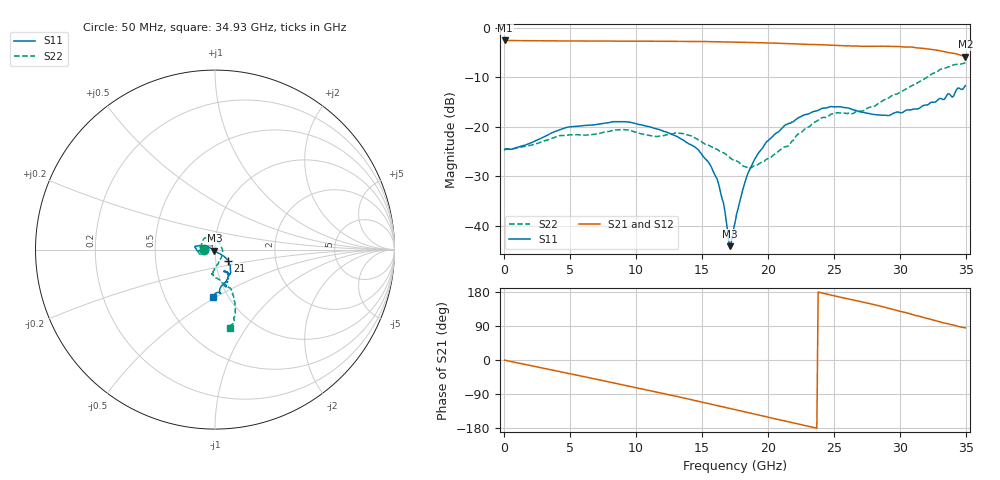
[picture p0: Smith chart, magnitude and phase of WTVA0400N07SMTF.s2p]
! 50 ohm 2-Port S-parameters measured by Modelithics Inc support@modelithics.com  Tampa, FL USA 813-866-6335 (February 2024)
! Smiths Interconnect,  4dB P/N: WTVA0400N07SMTF, Temperature: 125 C
! Board: 10 mil Rogers 4350B, Mounting Pad Dimensions: Length: 15 mils, Width: 25 mils, Gap: 40 mils.
# Hz S RI R 50
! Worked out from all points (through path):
!   352 points, 50 MHz to 34.93 GHz, reference 50 ohm
!   highest |S21| = -2.54 dB at 100 MHz (marker M1); lowest = -5.8 dB at 34.93 GHz (marker M2)
!   group delay of S21, straight-line fit = 21.8 ps
!   lowest |S11| = -44.1 dB at 17.11 GHz (marker M3), VSWR 1.01, Z = 49.6 - j0.508 ohm
!   |S11| at or under -10 dB: start of sweep to end of sweep
!   |S22| runs from -28.4 to -7.0 dB; largest |S21 - S12| = 0.0081
!   S11 on the Smith chart (normalised r, x): 50 MHz: 0.89, +0.00; 21 GHz: 1.15, -0.14; 34.93 GHz: 0.86, -0.48
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5e7  -0.0588 0.000987  0.7465 -0.00455  0.7458 -0.00454  -0.0589 -0.000771
1e8  -0.0595 0.000102  0.7465 -0.0101  0.7458 -0.0102  -0.0599 -0.000775
5.8715e9  -0.1026 -0.00105  0.5429 -0.4988  0.5423 -0.4983  -0.0763 -0.0317
9.155e9  -0.1116 0.0181  0.2924 -0.6738  0.2918 -0.6729  -0.093 -0.0108
1.1742e10  -0.0919 0.0211  0.0529 -0.7308  0.0514 -0.73  -0.0728 0.0348
1.44285e10  -0.0607 0.0172  -0.21 -0.6993  -0.2117 -0.6978  -0.0392 0.0674
1.56225e10  -0.039 0.0131  -0.3196 -0.6516  -0.3207 -0.6499  -0.00976 0.0634
1.612e10  -0.0287 0.00913  -0.3624 -0.6275  -0.3628 -0.6262  0.00126 0.0594
1.66175e10  -0.0164 0.00443  -0.4026 -0.5997  -0.4033 -0.5983  0.0115 0.0537
1.7115e10  -0.00361 -0.00511  -0.4417 -0.5693  -0.442 -0.5679  0.0189 0.045
1.7513e10  0.00247 -0.0109  -0.4724 -0.543  -0.4721 -0.5418  0.023 0.0393
1.8309e10  0.0213 -0.0206  -0.5259 -0.4832  -0.5254 -0.4823  0.0335 0.021
1.8906e10  0.035 -0.0288  -0.5605 -0.4365  -0.5601 -0.4352  0.0397 0.00651
2.09955e10  0.0734 -0.0615  -0.6504 -0.2492  -0.6495 -0.2488  0.0317 -0.0507
2.33835e10  0.086 -0.1135  -0.6791 -0.028  -0.6782 -0.0283  -0.00309 -0.1088
2.5473e10  0.0801 -0.1384  -0.6434 0.1654  -0.6424 0.1651  -0.0171 -0.1372
2.71645e10  0.0648 -0.1249  -0.5801 0.2978  -0.5781 0.2994  -0.00387 -0.145
2.91545e10  0.0553 -0.118  -0.4706 0.4509  -0.4655 0.4543  0.054 -0.1901
3.21395e10  0.0705 -0.1539  -0.1969 0.5792  -0.1939 0.579  0.111 -0.3058
3.3632e10  0.0609 -0.2081  -0.0517 0.5615  -0.0471 0.5612  0.1059 -0.3906
3.39305e10  0.0497 -0.1937  -0.0283 0.5553  -0.0242 0.5545  0.1065 -0.404
3.49255e10  -0.0101 -0.2614  0.0452 0.5088  0.0454 0.5076  0.0852 -0.4365
